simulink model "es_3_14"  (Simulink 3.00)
settings: Solver=ode1  SolverMode=SingleTasking  StartTime=0.0  StopTime=5  FixedStep=0.001  MaxStep=0.001  RelTol=1e-6  AbsTol=1e-6
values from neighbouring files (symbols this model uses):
  a = [0.5; 0.5; 0.5]    [inizia.M]
  Tc = 0.001    [inizia.M]
  Ts = @2;', 		'Mask Help','Implements a zeroth order discrete\nintegration using a gain, a sum, and\na unit delay. Inputs may be scalar\nor vector.\n')    [es_3_15.m]    (also in es_3_14.m; inizia.M = 0.002)

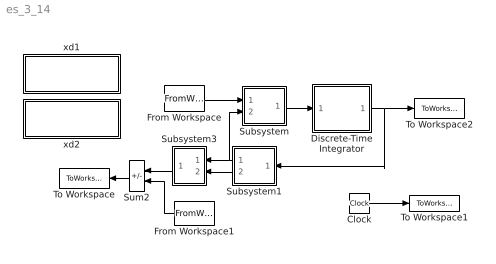
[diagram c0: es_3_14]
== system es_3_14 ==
  Clock : Clock
  Discrete-Time Integrator : Subsystem  mask(Discrete-Time Integrator){}
      mask help: Discrete-Time Integrator:
      mask init:
      | X0=@1;Ts=@2;
  From Workspace : FromWorkspace  VariableName=[T,dxd]  SampleTime=Tc  HoldFinalValue=off
  From Workspace1 : FromWorkspace  Orientation=left  VariableName=[T,xd]  SampleTime=Tc  HoldFinalValue=off
  Subsystem : Subsystem
  Subsystem1 : Subsystem  Orientation=left
  Subsystem3 : Subsystem  Orientation=left
  Sum2 : Sum  Orientation=left  Inputs=-+  SaturateOnIntegerOverflow=on
  To Workspace : ToWorkspace  VariableName=err  SampleTime=Ts  SaveFormat=Matrix
  To Workspace1 : ToWorkspace  VariableName=time  SampleTime=Ts  SaveFormat=Matrix
  To Workspace2 : ToWorkspace  VariableName=qout  SampleTime=Ts  SaveFormat=Matrix
  xd1 : Subsystem
  xd2 : Subsystem
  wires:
  Subsystem1/2(out_4) -> Subsystem3/2(iin_5)
  Subsystem1/1(out_5) -> Subsystem/2(in_2), Subsystem3/1(iin_4)
  Subsystem3/1(out_1) -> Sum2/1
  From Workspace1/1 -> Sum2/2
  Clock/1 -> To Workspace1/1
  Sum2/1 -> To Workspace/1
  Subsystem/1(out_1) -> Discrete-Time Integrator/1(in_1)
  Discrete-Time Integrator/1(out_1) -> To Workspace2/1, Subsystem1/1(in_1)
  From Workspace/1 -> Subsystem/1(in_1)

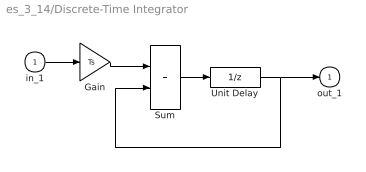
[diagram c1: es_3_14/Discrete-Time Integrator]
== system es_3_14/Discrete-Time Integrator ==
  in_1 : Inport  Port=1  PortWidth=-1  SampleTime=-1  DataType=auto
  Gain : Gain  Gain=Ts  SaturateOnIntegerOverflow=on
  Sum : Sum  Inputs=++  SaturateOnIntegerOverflow=on
  Unit Delay : UnitDelay  X0=X0  SampleTime=Ts
  out_1 : Outport  Port=1  InitialOutput=0
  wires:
  Gain/1 -> Sum/1
  in_1/1 -> Gain/1
  Sum/1 -> Unit Delay/1
  Unit Delay/1 -> out_1/1, Sum/2

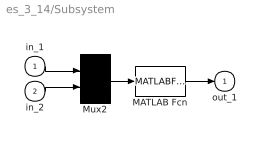
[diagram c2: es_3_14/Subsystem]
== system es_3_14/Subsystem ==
  in_1 : Inport  Port=1  PortWidth=-1  SampleTime=-1  DataType=auto
  in_2 : Inport  Port=2  PortWidth=-1  SampleTime=-1  DataType=auto
  MATLAB Fcn : MATLABFcn  MATLABFcn=invJa  OutputWidth=3  OutputSignalType=auto
  Mux2 : Mux  Inputs=[3,6]
  out_1 : Outport  Port=1  InitialOutput=0
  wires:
  Mux2/1 -> MATLAB Fcn/1
  in_1/1 -> Mux2/1
  MATLAB Fcn/1 -> out_1/1
  in_2/1 -> Mux2/2

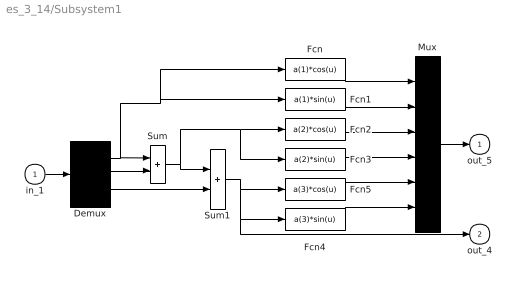
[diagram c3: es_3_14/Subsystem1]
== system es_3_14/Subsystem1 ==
  in_1 : Inport  Port=1  PortWidth=-1  SampleTime=-1  DataType=auto
  Demux : Demux  Outputs=3
  Fcn : Fcn  Expr=a(1)*cos(u)
  Fcn1 : Fcn  Expr=a(1)*sin(u)
  Fcn2 : Fcn  Expr=a(2)*cos(u)
  Fcn3 : Fcn  Expr=a(2)*sin(u)
  Fcn4 : Fcn  Expr=a(3)*sin(u)
  Fcn5 : Fcn  Expr=a(3)*cos(u)
  Mux : Mux  Inputs=6
  Sum : Sum  Inputs=++  SaturateOnIntegerOverflow=on
  Sum1 : Sum  Inputs=++  SaturateOnIntegerOverflow=on
  out_5 : Outport  Port=1  InitialOutput=0
  out_4 : Outport  Port=2  InitialOutput=0
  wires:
  in_1/1 -> Demux/1
  Demux/2 -> Sum/2
  Demux/3 -> Sum1/2
  Demux/1 -> Sum/1, Fcn/1, Fcn1/1
  Fcn/1 -> Mux/1
  Fcn1/1 -> Mux/2
  Fcn2/1 -> Mux/3
  Fcn3/1 -> Mux/4
  Fcn5/1 -> Mux/5
  Fcn4/1 -> Mux/6
  Sum1/1 -> Fcn5/1, Fcn4/1, out_4/1
  Mux/1 -> out_5/1
  Sum/1 -> Sum1/1, Fcn2/1, Fcn3/1

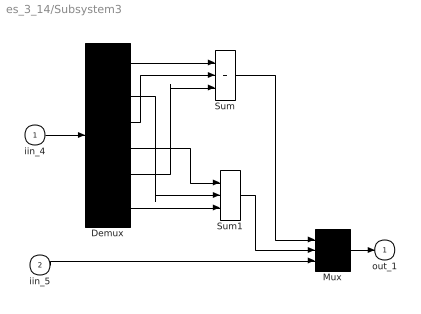
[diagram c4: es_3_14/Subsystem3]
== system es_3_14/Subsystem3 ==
  iin_4 : Inport  Port=1  PortWidth=-1  SampleTime=-1  DataType=auto
  iin_5 : Inport  Port=2  PortWidth=-1  SampleTime=-1  DataType=auto
  Demux : Demux  Outputs=6
  Mux : Mux  Inputs=3
  Sum : Sum  Inputs=+++  SaturateOnIntegerOverflow=on
  Sum1 : Sum  Inputs=+++  SaturateOnIntegerOverflow=on
  out_1 : Outport  Port=1  InitialOutput=0
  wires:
  iin_4/1 -> Demux/1
  Demux/1 -> Sum/1
  Demux/3 -> Sum/2
  Demux/5 -> Sum/3
  Demux/6 -> Sum1/3
  Demux/2 -> Sum1/2
  Demux/4 -> Sum1/1
  Sum1/1 -> Mux/2
  iin_5/1 -> Mux/3
  Sum/1 -> Mux/1
  Mux/1 -> out_1/1

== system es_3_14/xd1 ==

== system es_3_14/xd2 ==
